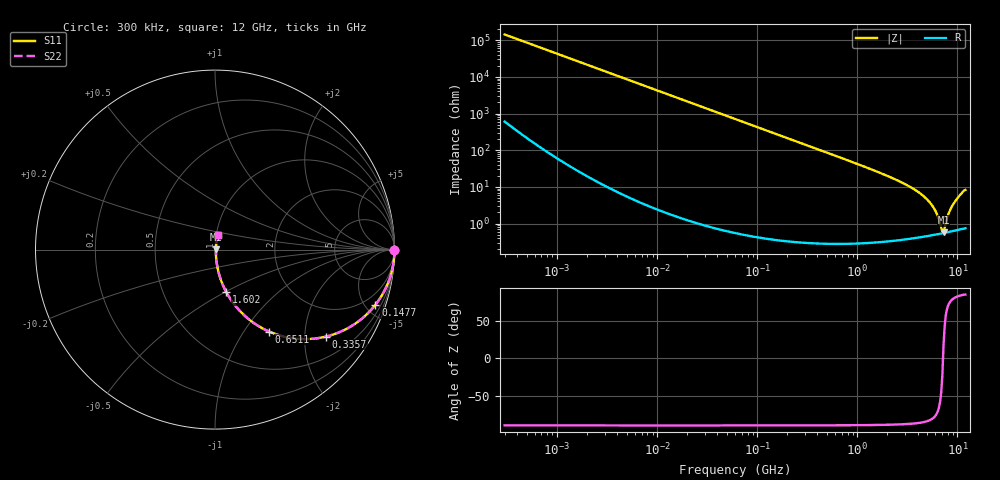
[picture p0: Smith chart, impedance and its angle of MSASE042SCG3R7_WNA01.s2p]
! MSASE042SCG3R7_WNA01  S-PARAMETER MODEL  ( General Type )
! Model Generated by TAIYO YUDEN Corporation (http://www.ty-top.com)
! Version 1.0
! TAIYO YUDEN Control No. 130801
! Copyright(c) 2013 TAIYO YUDEN CO.,LTD. All Rights Reserved.
! Product Description (link to TY-COMPAS)
! https://ds.yuden.co.jp/TYCOMPAS/or/detail?pn=MSASE042SCG3R7BWNA01&u=M
! Products Name : Multilayer Ceramic Capacitors
! Characteristics :
!  Capacitance : 3.7 pF , Rated Voltage : 16V , TCC : CG / C0G
!  Case Size : 0.4 x 0.2 / 0.016 x 0.008 [mm/inch] , Thickness : 0.2 / 0.008 [mm/inch]
!  (Conditions: Temperature = 25 degC , DC Bias Current/Voltage = 0A / 0V)
! External Node Assignments :
!  1  o---| |---o  2
! GND o---------o GND
! Frequency Range : 0.3MHz  -  12000MHz  [ 401 STEP ]
# MHz S RI R 50
! Freq[MHz].  S11 Real  S11 Imag  S21 Real  S21 Imag  S12 Real  S12 Imag  S22 Real  S22 Imag
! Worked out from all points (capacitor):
!   401 points, 300 kHz to 12 GHz, reference 50 ohm
!   read as one part in series: C = 3.71 pF near 316.3 kHz
!   lowest |Z| = 573 mohm at 7.254 GHz (marker M1)
!   series resonance near 7.176 GHz, so ESL is about 130 pH
!   S11 on the Smith chart (normalised r, x): 300 kHz: open; 147.7 MHz: 1.01, -5.81; 335.7 MHz: 1.01, -2.55; 651.1 MHz: 1.01, -1.31; 1.602 GHz: 1.01, -0.51; 12 GHz: 1.01, +0.16
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0.3  1 -0.000699  3.43e-06 0.000699  3.43e-06 0.000699  1 -0.000699
1.769972  1 -0.00412  2.1e-05 0.00412  2.1e-05 0.00412  1 -0.00412
10.44266  0.9994 -0.0243  0.000605 0.0243  0.000605 0.0243  0.9994 -0.0243
60  0.9808 -0.137  0.0192 0.137  0.0192 0.137  0.9808 -0.137
147.6816  0.8939 -0.3074  0.1061 0.3074  0.1061 0.3074  0.8939 -0.3074
335.7268  0.6194 -0.4844  0.3806 0.4844  0.3806 0.4844  0.6194 -0.4844
353.9943  0.594 -0.4899  0.406 0.4899  0.406 0.4899  0.594 -0.4899
651.0506  0.3005 -0.4564  0.6995 0.4564  0.6995 0.4564  0.3005 -0.4564
994.7115  0.1538 -0.3574  0.8462 0.3574  0.8462 0.3574  0.1538 -0.3574
1602.47  0.0635 -0.2379  0.9365 0.2379  0.9365 0.2379  0.0635 -0.2379
2088.533  0.0372 -0.1808  0.9628 0.1808  0.9628 0.1808  0.0372 -0.1808
3454.93  0.0128 -0.0941  0.9872 0.0941  0.9872 0.0941  0.0128 -0.0941
4875.354  0.00671 -0.0473  0.9933 0.0473  0.9933 0.0473  0.00671 -0.0473
5868.704  0.00548 -0.0244  0.9945 0.0244  0.9945 0.0244  0.00548 -0.0244
6354.153  0.00531 -0.0149  0.9947 0.0149  0.9947 0.0149  0.00531 -0.0149
6879.757  0.00534 -0.00549  0.9947 0.00549  0.9947 0.00549  0.00534 -0.00549
7254.098  0.00546 0.00162  0.9945 -0.00162  0.9945 -0.00162  0.00546 0.00162
7448.838  0.00557 0.00501  0.9944 -0.00501  0.9944 -0.00501  0.00557 0.00501
8281.503  0.00627 0.0196  0.9937 -0.0196  0.9937 -0.0196  0.00627 0.0196
8966.534  0.00712 0.0309  0.9929 -0.0309  0.9929 -0.0309  0.00712 0.0309
10511.28  0.01 0.0568  0.99 -0.0568  0.99 -0.0568  0.01 0.0568
12000  0.014 0.0805  0.986 -0.0805  0.986 -0.0805  0.014 0.0805
